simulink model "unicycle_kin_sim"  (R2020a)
settings: Solver=FixedStepAuto  StartTime=0.0  StopTime=inf  FixedStep=1e-4  RelTol=1e-3
undefined symbols (not defined in the file or in its folder): Clock, clock, cmd_vel, geometry_msgs, nav_msgs, odom, Odometry, rosgraph_msgs, tf2_msgs, TFMessage, Twist
libraries: robotlib x7

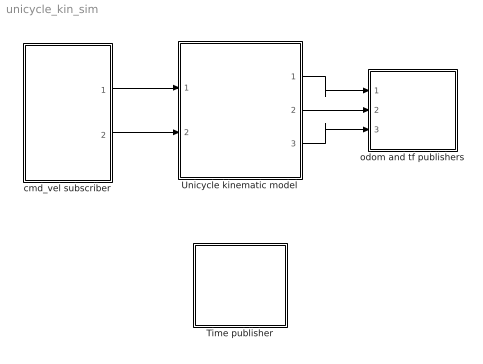
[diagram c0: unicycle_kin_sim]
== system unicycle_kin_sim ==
  Time publisher : Subsystem
  Unicycle kinematic model : Subsystem  mask{state0=[0,0,0]}
      mask prompts: state0 "Initial conditions (x0, y0, theta0)"
  cmd_vel subscriber : Subsystem
  odom and tf publishers : Subsystem  mask{simPublishRate=100}
      mask prompts: simPublishRate "Publising rate [Hz]"
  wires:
  Unicycle kinematic model/1(x) -> odom and tf publishers/1(x)
  Unicycle kinematic model/2(y) -> odom and tf publishers/2(y)
  Unicycle kinematic model/3(theta) -> odom and tf publishers/3(theta)
  cmd_vel subscriber/1(v) -> Unicycle kinematic model/1(v)
  cmd_vel subscriber/2(omega) -> Unicycle kinematic model/2(omega)

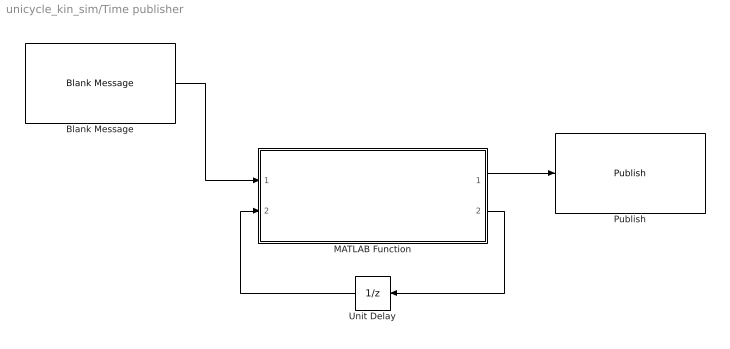
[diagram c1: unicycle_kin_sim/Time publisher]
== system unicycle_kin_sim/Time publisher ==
  Blank Message : robotlib/Blank Message  messageClass=Message  entityType=rosgraph_msgs/Clock  messageType=rosgraph_msgs/Clock  SampleTime=1e-4
  MATLAB Function : MATLAB Function  TreatAsAtomicUnit=on
  Publish : robotlib/Publish  topicSource=Specify your own  topic=/clock  messageType=rosgraph_msgs/Clock  messageQueueLength=1
  Unit Delay : UnitDelay  SampleTime=1e-4  HasFrameUpgradeWarning=on
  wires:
  MATLAB Function/1(timeMsg) -> Publish/1
  Blank Message/1 -> MATLAB Function/1(blankMsg)
  MATLAB Function/2(count) -> Unit Delay/1
  Unit Delay/1 -> MATLAB Function/2(count_prev)

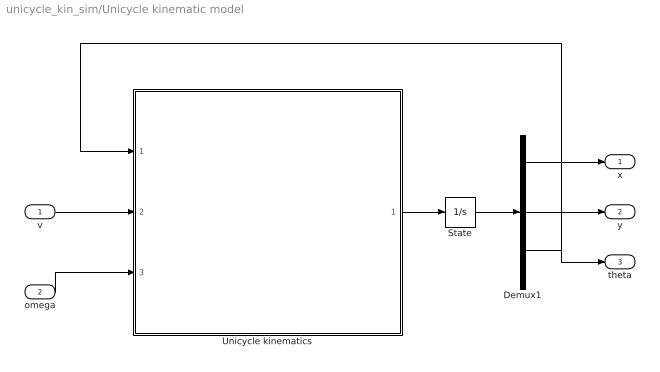
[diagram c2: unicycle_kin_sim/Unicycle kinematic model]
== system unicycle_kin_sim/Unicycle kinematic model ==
  v : Inport
  omega : Inport  Port=2
  Demux1 : Demux  Outputs=3
  State : Integrator  InitialCondition=state0
  Unicycle kinematics : MATLAB Function  TreatAsAtomicUnit=on
  x : Outport  VectorParamsAs1DForOutWhenUnconnected=off
  y : Outport  Port=2  VectorParamsAs1DForOutWhenUnconnected=off
  theta : Outport  Port=3  VectorParamsAs1DForOutWhenUnconnected=off
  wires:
  Demux1/3 -> Unicycle kinematics/1(theta), theta/1
  Unicycle kinematics/1(dstate) -> State/1
  State/1 -> Demux1/1
  Demux1/2 -> y/1
  Demux1/1 -> x/1
  omega/1 -> Unicycle kinematics/3(omega)
  v/1 -> Unicycle kinematics/2(v)

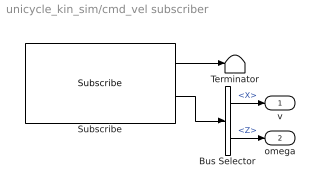
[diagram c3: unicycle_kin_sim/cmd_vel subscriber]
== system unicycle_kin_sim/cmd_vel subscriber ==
  Bus Selector : BusSelector  OutputSignals=Linear.X,Angular.Z
  Subscribe : robotlib/Subscribe  topicSource=Specify your own  topic=/cmd_vel  messageType=geometry_msgs/Twist  sampleTime=-1  messageQueueLength=1
  Terminator : Terminator
  v : Outport
  omega : Outport  Port=2
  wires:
  Bus Selector/1 -> v/1  "<X>"
  Subscribe/2 -> Bus Selector/1
  Subscribe/1 -> Terminator/1
  Bus Selector/2 -> omega/1  "<Z>"

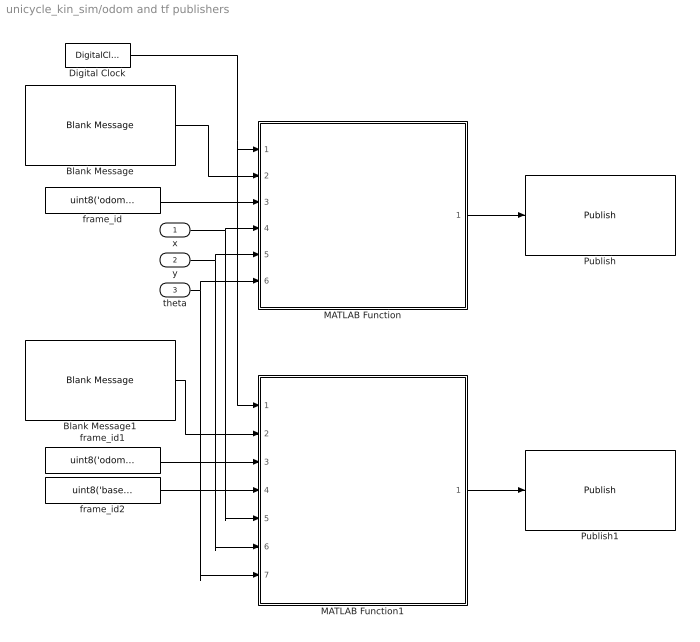
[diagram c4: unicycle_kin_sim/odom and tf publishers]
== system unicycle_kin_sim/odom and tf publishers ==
  x : Inport  SampleTime=1/simPublishRate
  y : Inport  Port=2  SampleTime=1/simPublishRate
  theta : Inport  Port=3  SampleTime=1/simPublishRate
  Blank Message : robotlib/Blank Message  messageClass=Message  entityType=nav_msgs/Odometry  messageType=nav_msgs/Odometry  SampleTime=1/simPublishRate
  Blank Message1 : robotlib/Blank Message  messageClass=Message  entityType=tf2_msgs/TFMessage  messageType=tf2_msgs/TFMessage  SampleTime=1/simPublishRate
  Digital Clock : DigitalClock  SampleTime=1/simPublishRate
  MATLAB Function : MATLAB Function  TreatAsAtomicUnit=on
  MATLAB Function1 : MATLAB Function  TreatAsAtomicUnit=on
  Publish : robotlib/Publish  topicSource=Specify your own  topic=/odom  messageType=nav_msgs/Odometry  messageQueueLength=1
  Publish1 : robotlib/Publish  topicSource=Specify your own  topic=/tf  messageType=tf2_msgs/TFMessage  messageQueueLength=1
  frame_id : Constant  Value=uint8('odom')
  frame_id1 : Constant  Value=uint8('odom')
  frame_id2 : Constant  Value=uint8('base_link')
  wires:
  MATLAB Function/1(odomMsg) -> Publish/1
  theta/1 -> MATLAB Function1/7(theta), MATLAB Function/6(theta)
  y/1 -> MATLAB Function/5(y), MATLAB Function1/6(y)
  x/1 -> MATLAB Function/4(x), MATLAB Function1/5(x)
  Blank Message/1 -> MATLAB Function/2(blankMsg)
  Digital Clock/1 -> MATLAB Function1/1(time), MATLAB Function/1(time)
  frame_id/1 -> MATLAB Function/3(frame_id)
  MATLAB Function1/1(tf2Msg) -> Publish1/1
  Blank Message1/1 -> MATLAB Function1/2(blankMsg)
  frame_id1/1 -> MATLAB Function1/3(targetFrame)
  frame_id2/1 -> MATLAB Function1/4(sourceFrame)

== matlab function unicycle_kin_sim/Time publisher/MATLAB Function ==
function [timeMsg,count] = generate_time_msg(blankMsg,count_prev)

time = count_prev*1e5;

blankMsg.Clock_.Sec = round(time*1e-9);
blankMsg.Clock_.Nsec = round(time-round(time));

count = count_prev+1;

timeMsg = blankMsg;

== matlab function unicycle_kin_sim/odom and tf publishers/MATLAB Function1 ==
function tf2Msg = generate_tf2_msg(time,blankMsg, targetFrame, sourceFrame, x, y, theta)

% Set the number of transforms
blankMsg.Transforms_SL_Info.CurrentLength = uint32(1);

% Writing transform header
blankMsg.Transforms(1).Header.Stamp.Sec = fix(time);
blankMsg.Transforms(1).Header.Stamp.Nsec = fix((time-fix(time))*1e9);
blankMsg.Transforms(1).Header.FrameId(1:length(targetFrame)) = targetFrame;
blankMsg.Transforms(1).Header.FrameId_SL_Info.CurrentLength = uint32(length(targetFrame));

blankMsg.Transforms(1).ChildFrameId(1:length(sourceFrame)) = sourceFrame;
blankMsg.Transforms(1).ChildFrameId_SL_Info.CurrentLength = uint32(length(sourceFrame));

% Writing transform traslation and rotation data
blankMsg.Transforms(1).Transform.Translation.X = x;
blankMsg.Transforms(1).Transform.Translation.Y = y;
blankMsg.Transforms(1).Transform.Translation.Z = 0;

rotation = eul2quat([0, 0, theta], 'ZYX');
blankMsg.Transforms(1).Transform.Rotation.X = rotation(1);
blankMsg.Transforms(1).Transform.Rotation.Y = rotation(2);
blankMsg.Transforms(1).Transform.Rotation.Z = rotation(3);
blankMsg.Transforms(1).Transform.Rotation.W = rotation(4);

tf2Msg = blankMsg;

== matlab function unicycle_kin_sim/Unicycle kinematic
model/Unicycle kinematics ==
function dstate = unicycle_kinematics(theta, v, omega)

dx     = v*cos(theta);
dy     = v*sin(theta);
dtheta = omega;

dstate = [dx, dy, dtheta];

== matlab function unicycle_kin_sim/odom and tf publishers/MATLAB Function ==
function odomMsg = generate_odom_msg(time,blankMsg,frame_id,x,y,theta)

% Writing the message header
blankMsg.Header.Stamp.Sec = fix(time);
blankMsg.Header.Stamp.Nsec = fix((time-fix(time))*1e9);
blankMsg.Header.FrameId(1:length(frame_id)) = frame_id;
blankMsg.Header.FrameId_SL_Info.CurrentLength = uint32(length(frame_id));

% Write pose data
blankMsg.Pose.Pose.Position.X = x;
blankMsg.Pose.Pose.Position.Y = y;
blankMsg.Pose.Pose.Position.Z = 0;

orientation = eul2quat([0, 0, theta], 'ZYX');
blankMsg.Pose.Pose.Orientation.X = orientation(1);
blankMsg.Pose.Pose.Orientation.Y = orientation(2);
blankMsg.Pose.Pose.Orientation.Z = orientation(3);
blankMsg.Pose.Pose.Orientation.W = orientation(4);

odomMsg = blankMsg;
